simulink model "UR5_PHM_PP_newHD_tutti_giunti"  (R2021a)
settings: Solver=ode14x  StartTime=0.0  StopTime=Sim.time  FixedStep=Sim.dt  MaxStep=Sim.dt  RelTol=1e-3  EnableMultiTasking=on
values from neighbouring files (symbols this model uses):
  alpha_n = 0.98*pi/180    (= 0.0171042266695)    [parameters.m]
  alpha_t = 30*pi/180    (= 0.523598775598)    [parameters.m]
  alpha_TTS = 0    [parameters.m]
  alpha_Tw_L = -6.9e-4    (= -0.00069)    [parameters.m]
  alpha_Tw_R = 3.9e-3    (= 0.0039)    [parameters.m]
  Beta_TTS = 0    [parameters.m]
  c1 = 1e-2    (= 0.01)    [parameters.m]
  c2 = 1e-2    (= 0.01)    [parameters.m]
  c3 = 1e-2    (= 0.01)    [parameters.m]
  c4 = 1e-2    (= 0.01)    [parameters.m]
  c5 = 1e-2    (= 0.01)    [parameters.m]
  c6 = 1e-2    (= 0.01)    [parameters.m]
  Cb1 = 1.8e3    (= 1800)    [parameters.m]
  Cb2 = 1.8e3    (= 1800)    [parameters.m]
  Cb3 = 1.8e3    (= 1800)    [parameters.m]
  Cb4 = 1.8e3    (= 1800)    [parameters.m]
  Cb5 = 1.8e3    (= 1800)    [parameters.m]
  Cb6 = 1.8e3    (= 1800)    [parameters.m]
  Cth_housing = 153.90    (= 153.9)    [parameters.m]
  Cth_w = 74.20    (= 74.2)    [parameters.m]
  dt_PP = 0.05    [parameters.m]
  Fric1 = [fc_1/2 1e1 fc_1 fv_1]    [parameters.m]
  Fric2 = [fc_2/2 1e1 fc_2 fv_2]    [parameters.m]
  Fric3 = [fc_3/2 1e1 fc_3 fv_3]    [parameters.m]
  Fric4 = [fc_4/2 1e1 fc_4 fv_4]    [parameters.m]
  Fric5 = [fc_5/2 1e1 fc_5 fv_5]    [parameters.m]
  Fric6 = [fc_6/2 1e1 fc_6 fv_6]    [parameters.m]
  Hth_housing = 0.30    (= 0.3)    [parameters.m]
  Hth_w = 1.14    [parameters.m]
  I_actual = I_actual(1:10,:)    [trajcutting.m]
  J_CS1 = 7.12e-5    (= 7.12e-05)    [parameters.m]
  J_CS2 = 7.12e-5    (= 7.12e-05)    [parameters.m]
  J_CS3 = 7.12e-5    (= 7.12e-05)    [parameters.m]
  J_CS4 = 6e-6    (= 6e-06)    [parameters.m]
  J_CS5 = 6e-6    (= 6e-06)    [parameters.m]
  J_CS6 = 6e-6    (= 6e-06)    [parameters.m]
  J_FS1 = 1.62e-7    (= 1.62e-07)    [parameters.m]
  J_FS2 = 1.62e-7    (= 1.62e-07)    [parameters.m]
  J_FS3 = 1.62e-7    (= 1.62e-07)    [parameters.m]
  J_FS4 = 4.97e-8    (= 4.97e-08)    [parameters.m]
  J_FS5 = 4.97e-8    (= 4.97e-08)    [parameters.m]
  J_FS6 = 4.97e-8    (= 4.97e-08)    [parameters.m]
  J_WG1 = 3.56e-5    (= 3.56e-05)    [parameters.m]
  J_WG2 = 3.56e-5    (= 3.56e-05)    [parameters.m]
  J_WG3 = 3.56e-5    (= 3.56e-05)    [parameters.m]
  J_WG4 = 3e-6    (= 3e-06)    [parameters.m]
  J_WG5 = 3e-6    (= 3e-06)    [parameters.m]
  J_WG6 = 3e-6    (= 3e-06)    [parameters.m]
  K_i = 1    [parameters.m]
  K_p = 1    [parameters.m]
  K_torsCS1 = 4.78e6    (= 4780000)    [parameters.m]
  K_torsCS2 = 4.78e6    (= 4780000)    [parameters.m]
  K_torsCS3 = 4.78e6    (= 4780000)    [parameters.m]
  K_torsCS4 = 1.06e6    (= 1060000)    [parameters.m]
  K_torsCS5 = 1.06e6    (= 1060000)    [parameters.m]
  K_torsCS6 = 1.06e6    (= 1060000)    [parameters.m]
  K_torsWG1 = 9.56e5    (= 956000)    [parameters.m]
  K_torsWG2 = 9.56e5    (= 956000)    [parameters.m]
  K_torsWG3 = 9.56e5    (= 956000)    [parameters.m]
  K_torsWG4 = 1.84e5    (= 184000)    [parameters.m]
  K_torsWG5 = 1.84e5    (= 184000)    [parameters.m]
  K_torsWG6 = 1.84e5    (= 184000)    [parameters.m]
  K_v = 1    [parameters.m]
  Kb1 = 0.51e8    (= 51000000)    [parameters.m]
  Kb2 = 0.51e8    (= 51000000)    [parameters.m]
  Kb3 = 0.51e8    (= 51000000)    [parameters.m]
  Kb4 = 1.98e7    (= 19800000)    [parameters.m]
  Kb5 = 1.98e7    (= 19800000)    [parameters.m]
  Kb6 = 1.98e7    (= 19800000)    [parameters.m]
  Km1 = 1.2e9    (= 1200000000)    [parameters.m]
  Km2 = 1.2e9    (= 1200000000)    [parameters.m]
  Km3 = 1.2e9    (= 1200000000)    [parameters.m]
  Km4 = 5.55e8    (= 555000000)    [parameters.m]
  Km5 = 5.55e8    (= 555000000)    [parameters.m]
  Km6 = 5.55e8    (= 555000000)    [parameters.m]
  Kt1 = 0.96e5    (= 96000)    [parameters.m]
  Kt2 = 0.96e5    (= 96000)    [parameters.m]
  Kt3 = 0.96e5    (= 96000)    [parameters.m]
  Kt4 = 1.15e4    (= 11500)    [parameters.m]
  Kt5 = 1.15e4    (= 11500)    [parameters.m]
  Kt6 = 1.15e4    (= 11500)    [parameters.m]
  L = Motor.L_2/2    [parameters.m]
  m2 = polyfit(Temp(:,2),pBn_UR5_f_Temp(:,2),1)    [parameters.m]
  mb2 = polyfit(Temp(:,8),pBn_UR5_f_Temp(:,8),1)    [parameters.m]
  pickTime = t_pick(traj)    [parameters.m]
  placeTime = t_place(traj)    [parameters.m]
  q0 = q_target(1,:)    [testlaw_PP.m]
  q_CS01 = x(6)    [parameters.m]
  q_CS02 = x(6)    [parameters.m]
  q_CS03 = x(6)    [parameters.m]
  q_CS04 = x(6)    [parameters.m]
  q_CS05 = x(6)    [parameters.m]
  q_CS06 = x(6)    [parameters.m]
  q_WG01 = x(1)    [parameters.m]
  q_WG02 = x(1)    [parameters.m]
  q_WG03 = x(1)    [parameters.m]
  q_WG04 = x(1)    [parameters.m]
  q_WG05 = x(1)    [parameters.m]
  q_WG06 = x(1)    [parameters.m]
  quant_i = [Motor.imax1 Motor.imax2      Motor.imax3 Motor.imax4 Motor.imax5 Motor.imax6]/2^16    [parameters.m]
  R = Motor.R_2/2    [parameters.m]
  rg1 = 0.028    [parameters.m]
  rg2 = 0.028    [parameters.m]
  rg3 = 0.028    [parameters.m]
  rg4 = 0.0155    [parameters.m]
  rg5 = 0.0155    [parameters.m]
  rg6 = 0.0155    [parameters.m]
  sigma_p = 444.29    [parameters.m]
  sigma_v = 2*pi*1000    (= 6283.18530718)    [parameters.m]
  stiff_red = 1    [parameters.m]
  T_0 = Sim.temp    [parameters.m]
  T_switch = 1e-4    (= 0.0001)    [parameters.m]
  tau_i = 1/(fc_i*2*pi)    (= 7.95774715459e-05)    [parameters.m]
  U_s = 48    [parameters.m]
  var_i = 1e-1*[.0167 .0184 .0144 .0016      .0011 .0007]    [parameters.m]
  var_p = 1e-6*[.0943 .3877      .3478 .5436 .3400 .2081]    [parameters.m]
  var_v = 1e-4*[.0738 .1452      .1564 .4623 .1824 .0917]    [parameters.m]
  Wf_TTS_0 = 0    [parameters.m]
  Wf_TTS_ONOFF = 0    [parameters.m]
  x2_01 = x(3)    [parameters.m]
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undefined symbols (not defined in the file or in its folder): deg, Driver1, Driver2, Driver3, Driver4, Driver5, Driver6, elseif, geom, Ground, J1, J2, J3, J4, J5, J6, kg, L1, L2, L3, L4, L5, L6, LINK0, LINK1, LINK2, LINK3, LINK4, LINK5, LINK6, m, Motor, N, payload, ROBOTIQ_FT, s, Sim, Tool, X, Y, Z
libraries: sm_lib x35, nesl_utility x30, simulink x23, simulink_extras x11, spsTriangleGeneratorLib x6
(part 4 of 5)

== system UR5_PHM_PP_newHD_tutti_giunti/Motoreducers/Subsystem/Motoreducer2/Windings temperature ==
  note: Coupling
  note: Housing
  note: Windings
  note: W_joule
  W_joule [W] : Inport
  T_ext [°C] : Inport  Port=2
  Add : Sum  Inputs=-+
  Add1 : Sum  Inputs=+-
  Add2 : Sum  Inputs=+-
  Add3 : Sum  Inputs=-+
  Add4 : Sum  Inputs=+-
  Gain : Gain  Gain=Hth_housing
  Gain1 : Gain  Gain=1/Cth_w
  Gain2 : Gain  Gain=Hth_w
  Gain3 : Gain  Gain=1/Cth_housing
  Gain4 : Gain  Gain=Hth_housing
  Integrator : Integrator  InitialCondition=T_0  LimitOutput=on  LowerSaturationLimit=-273.15
  Integrator1 : Integrator  InitialCondition=T_0  LimitOutput=on  LowerSaturationLimit=-273.15
  Tw [°C] : Outport  VectorParamsAs1DForOutWhenUnconnected=off
  Th [°C] : Outport  Port=2
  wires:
  W_joule [W]/1 -> Add/2
  Add/1 -> Gain1/1
  Gain1/1 -> Integrator/1
  Gain2/1 -> Add/1
  Integrator/1 -> Add2/1, Add1/1, Tw [°C]/1  "Tw"
  Add2/1 -> Gain2/1
  Integrator1/1 -> Th [°C]/1, Add3/2, Add1/2, Add2/2  "Thouse"
  Gain3/1 -> Integrator1/1
  T_ext [°C]/1 -> Add3/1
  Add1/1 -> Gain/1
  Add3/1 -> Gain4/1
  Gain4/1 -> Add4/2
  Gain/1 -> Add4/1
  Add4/1 -> Gain3/1

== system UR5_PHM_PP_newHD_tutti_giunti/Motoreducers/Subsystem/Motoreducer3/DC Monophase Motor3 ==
  Vset : Inport
  C : Inport  Port=2
  Gain4 : Gain  Gain=1/Motor.Im_123
  Integrator : Integrator
  Integrator1 : Integrator  InitialCondition=q0(3)*Motor.tau
  Monophase - BLDC : Subsystem
  Mux : Mux  Inputs=3
  Sum : Sum  Inputs=|+-
  i : Outport
  qm,qdm,qddm : Outport  Port=2  VectorParamsAs1DForOutWhenUnconnected=off
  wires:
  Monophase - BLDC/2(i) -> i/1  "i_j3"
  Vset/1 -> Monophase - BLDC/1(Vset)
  Monophase - BLDC/1(T) -> Sum/1  "Tem_j3"
  Sum/1 -> Gain4/1  "Tem-C_j3"
  Gain4/1 -> Mux/3, Integrator/1
  Integrator/1 -> Monophase - BLDC/2(qdm), Mux/2, Integrator1/1
  Mux/1 -> qm,qdm,qddm/1
  Integrator1/1 -> Mux/1  "qm_j3"
  C/1 -> Sum/2  "C_j3"

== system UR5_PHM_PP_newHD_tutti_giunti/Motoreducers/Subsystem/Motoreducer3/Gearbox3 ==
  C : Inport
  qd : Inport  Port=2
  " eta" : Gain  Gain=Motor.eta
  Abs : Abs
  Abs2 : Abs
  Add2 : Sum  Inputs=+|-
  Friction Function1 : Fcn  Expr=Fric3(1)*(1-tanh(Fric3(2)*u)) + Fric3(3) + Fric3(4)*u
  MinMax2 : MinMax  Inputs=2
  Product : Product  RndMeth=Zero
  Saturation : Saturate  UpperLimit=150  LowerLimit=-150
  Sign : Signum
  Sign1 : Signum
  Switch : Switch  Criteria=u2 > Threshold  Threshold=0.0
  Switch1 : Switch  Criteria=u2 > Threshold  Threshold=0.5
  Zero Detection : Fcn  Expr=abs(u(1))<1e-6
  Tu : Outport  VectorParamsAs1DForOutWhenUnconnected=off
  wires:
  Friction Function1/1 -> MinMax2/2, Switch1/3
  Add2/1 -> Tu/1  "Transmitted torque [Nm]"
  Zero Detection/1 -> Switch/2, Switch1/2
  C/1 -> " eta"/1
  Sign1/1 -> Switch/3
  " eta"/1 -> Saturation/1
  Switch1/1 -> Product/2
  Abs2/1 -> Friction Function1/1
  Sign/1 -> Switch/1
  Product/1 -> Add2/2  "Passive torque [Nm]"
  Switch/1 -> Product/1
  qd/1 -> Zero Detection/1, Sign1/1, Abs2/1
  MinMax2/1 -> Switch1/1
  Abs/1 -> MinMax2/1
  Saturation/1 -> Sign/1, Abs/1, Add2/1

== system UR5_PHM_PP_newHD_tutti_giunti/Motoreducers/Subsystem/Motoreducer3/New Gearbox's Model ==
  Delta_q : Inport
  qm : Inport  Port=2
  qdm : Inport  Port=3
  Delta_qd : Inport  Port=4
  q : Inport  Port=5
  qd : Inport  Port=6
  Abs : Abs
  Constant1 : Constant  Value=0
  Constant2 : Constant  Value=J3.clearance
  Constant3 : Constant  Value=J3.clearance
  Mux : Mux  Inputs=3
  No Backlash : Subsystem  TreatAsAtomicUnit=on
  No contact : Subsystem  Commented=on  TreatAsAtomicUnit=on
  Scope : Scope
  "if Height < Max low altitude elseif Height > Min isotropic altitude " : If  NumInputs=4  IfExpression=u1<=1e-10  ElseIfExpressions=u2>u3, u2<u4
  phi diff > max backlash : Subsystem  Commented=on  TreatAsAtomicUnit=on
  phi diff< min backlash : Subsystem  Commented=on  TreatAsAtomicUnit=on
  C1 : Outport
  Tu : Outport  Port=2  VectorParamsAs1DForOutWhenUnconnected=off
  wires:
  Constant3/1 -> Abs/1
  [Vel_rel] -> No contact/2(In3)
  [Pos_rel] -> No contact/1(In2)
  No contact/1(Out3) -> ?
  [ELSE] -> No contact/Action
  phi diff< min backlash/1(Out1) -> ?
  phi diff > max backlash/1(Out1) -> ?
  [Pos_rel] -> phi diff< min backlash/1(In2)
  [Vel_rel] -> phi diff< min backlash/2(In3)
  [ELSEIF2] -> phi diff< min backlash/Action
  [Pos_rel] -> phi diff > max backlash/1(In2)
  [Vel_rel] -> phi diff > max backlash/2(In3)
  [IF] -> No Backlash/Action
  [ELSEIF1] -> phi diff > max backlash/Action
  "if Height < Max low altitude elseif Height > Min isotropic altitude "/3 -> [ELSEIF2]
  Constant1/1 -> Mux/3, "if Height < Max low altitude elseif Height > Min isotropic altitude "/4
  Constant2/1 -> Mux/2, "if Height < Max low altitude elseif Height > Min isotropic altitude "/3
  Abs/1 -> "if Height < Max low altitude elseif Height > Min isotropic altitude "/1
  "if Height < Max low altitude elseif Height > Min isotropic altitude "/4 -> [ELSE]
  "if Height < Max low altitude elseif Height > Min isotropic altitude "/2 -> [ELSEIF1]
  "if Height < Max low altitude elseif Height > Min isotropic altitude "/1 -> [IF]
  Delta_q/1 -> Mux/1, "if Height < Max low altitude elseif Height > Min isotropic altitude "/2, [Pos_rel]
  Mux/1 -> Scope/1
  Delta_qd/1 -> [Vel_rel]
  No Backlash/1(Ccs->giunto) -> Tu/1
  q/1 -> No Backlash/2(q)
  qm/1 -> No Backlash/1(qm)
  qdm/1 -> No Backlash/3(qdm)
  qd/1 -> No Backlash/4(qd)
  No Backlash/2(Cwg->rotore) -> C1/1

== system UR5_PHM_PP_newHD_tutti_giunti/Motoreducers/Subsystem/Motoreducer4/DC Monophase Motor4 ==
  Vset : Inport
  C : Inport  Port=2
  Gain4 : Gain  Gain=1/Motor.Im_456
  Integrator : Integrator
  Integrator1 : Integrator  InitialCondition=q0(4)*Motor.tau
  Monophase - BLDC : Subsystem
  Mux : Mux  Inputs=3
  Sum : Sum  Inputs=|+-
  i : Outport
  qm,qdm,qddm : Outport  Port=2  VectorParamsAs1DForOutWhenUnconnected=off
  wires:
  Monophase - BLDC/2(i) -> i/1  "i_j4"
  Vset/1 -> Monophase - BLDC/1(Vset)
  Monophase - BLDC/1(T) -> Sum/1  "Tem_j4"
  Sum/1 -> Gain4/1  "Tem-C_j4"
  Gain4/1 -> Mux/3, Integrator/1
  Integrator/1 -> Monophase - BLDC/2(qdm), Mux/2, Integrator1/1
  Mux/1 -> qm,qdm,qddm/1
  Integrator1/1 -> Mux/1  "qm_j4"
  C/1 -> Sum/2  "C_j4"

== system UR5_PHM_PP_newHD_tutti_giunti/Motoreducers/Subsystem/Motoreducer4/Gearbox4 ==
  C : Inport
  qd : Inport  Port=2
  " eta" : Gain  Gain=Motor.eta
  Abs : Abs
  Abs2 : Abs
  Add2 : Sum  Inputs=+|-
  Friction Function1 : Fcn  Expr=Fric4(1)*(1-tanh(Fric4(2)*u)) + Fric4(3) + Fric4(4)*u
  MinMax2 : MinMax  Inputs=2
  Product : Product  RndMeth=Zero
  Saturation : Saturate  UpperLimit=28  LowerLimit=-28
  Sign : Signum
  Sign1 : Signum
  Switch : Switch  Criteria=u2 > Threshold  Threshold=0.0
  Switch1 : Switch  Criteria=u2 > Threshold  Threshold=0.5
  Zero Detection : Fcn  Expr=abs(u(1))<1e-6
  Tu : Outport  VectorParamsAs1DForOutWhenUnconnected=off
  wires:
  Switch1/1 -> Product/2
  Sign/1 -> Switch/1
  Product/1 -> Add2/2  "Passive torque [Nm]"
  Switch/1 -> Product/1
  C/1 -> " eta"/1
  MinMax2/1 -> Switch1/1
  Sign1/1 -> Switch/3
  Add2/1 -> Tu/1  "Transmitted torque [Nm]"
  Abs/1 -> MinMax2/1
  " eta"/1 -> Saturation/1
  Abs2/1 -> Friction Function1/1
  Friction Function1/1 -> MinMax2/2, Switch1/3
  Zero Detection/1 -> Switch/2, Switch1/2
  qd/1 -> Zero Detection/1, Sign1/1, Abs2/1
  Saturation/1 -> Sign/1, Abs/1, Add2/1

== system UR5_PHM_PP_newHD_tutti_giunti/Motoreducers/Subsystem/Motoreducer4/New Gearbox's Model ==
  Delta_q : Inport
  qm : Inport  Port=2
  qdm : Inport  Port=3
  Delta_qd : Inport  Port=4
  q : Inport  Port=5
  qd : Inport  Port=6
  Abs : Abs
  Constant1 : Constant  Value=0
  Constant2 : Constant  Value=J4.clearance
  Constant3 : Constant  Value=J4.clearance
  Mux : Mux  Inputs=3
  No Backlash : Subsystem  TreatAsAtomicUnit=on
  No contact : Subsystem  Commented=on  TreatAsAtomicUnit=on
  Scope : Scope
  "if Height < Max low altitude elseif Height > Min isotropic altitude " : If  NumInputs=4  IfExpression=u1<=1e-10  ElseIfExpressions=u2>u3, u2<u4
  phi diff > max backlash : Subsystem  Commented=on  TreatAsAtomicUnit=on
  phi diff< min backlash : Subsystem  Commented=on  TreatAsAtomicUnit=on
  C1 : Outport
  C2 : Outport  Port=2  VectorParamsAs1DForOutWhenUnconnected=off
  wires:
  Constant3/1 -> Abs/1
  [Vel_rel] -> No contact/2(In3)
  [Pos_rel] -> No contact/1(In2)
  No contact/1(Out3) -> ?
  [ELSE] -> No contact/Action
  phi diff< min backlash/1(Out1) -> ?
  phi diff > max backlash/1(Out1) -> ?
  [Pos_rel] -> phi diff< min backlash/1(In2)
  [Vel_rel] -> phi diff< min backlash/2(In3)
  [ELSEIF2] -> phi diff< min backlash/Action
  [Pos_rel] -> phi diff > max backlash/1(In2)
  [Vel_rel] -> phi diff > max backlash/2(In3)
  [IF] -> No Backlash/Action
  [ELSEIF1] -> phi diff > max backlash/Action
  "if Height < Max low altitude elseif Height > Min isotropic altitude "/3 -> [ELSEIF2]
  Constant1/1 -> Mux/3, "if Height < Max low altitude elseif Height > Min isotropic altitude "/4
  Constant2/1 -> Mux/2, "if Height < Max low altitude elseif Height > Min isotropic altitude "/3
  Abs/1 -> "if Height < Max low altitude elseif Height > Min isotropic altitude "/1
  "if Height < Max low altitude elseif Height > Min isotropic altitude "/4 -> [ELSE]
  "if Height < Max low altitude elseif Height > Min isotropic altitude "/2 -> [ELSEIF1]
  "if Height < Max low altitude elseif Height > Min isotropic altitude "/1 -> [IF]
  Delta_q/1 -> Mux/1, "if Height < Max low altitude elseif Height > Min isotropic altitude "/2, [Pos_rel]
  Mux/1 -> Scope/1
  Delta_qd/1 -> [Vel_rel]
  qm/1 -> No Backlash/1(qm)
  q/1 -> No Backlash/2(q)
  qdm/1 -> No Backlash/3(qdm)
  qd/1 -> No Backlash/4(qd)
  No Backlash/1(Ccs->giunto) -> C2/1
  No Backlash/2(Cwg->rotore) -> C1/1

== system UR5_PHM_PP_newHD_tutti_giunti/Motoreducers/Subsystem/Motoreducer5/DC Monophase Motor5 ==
  Vset : Inport
  C : Inport  Port=2
  Gain4 : Gain  Gain=1/Motor.Im_456
  Integrator : Integrator
  Integrator1 : Integrator  InitialCondition=q0(5)*Motor.tau
  Monophase - BLDC : Subsystem
  Mux : Mux  Inputs=3
  Sum : Sum  Inputs=|+-
  i : Outport
  qm,qdm,qddm : Outport  Port=2  VectorParamsAs1DForOutWhenUnconnected=off
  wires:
  Monophase - BLDC/2(i) -> i/1  "i_j5"
  Vset/1 -> Monophase - BLDC/1(Vset)
  Monophase - BLDC/1(T) -> Sum/1  "Tem_j5"
  Sum/1 -> Gain4/1  "Tem-C_j5"
  Gain4/1 -> Mux/3, Integrator/1
  Integrator/1 -> Monophase - BLDC/2(qdm), Mux/2, Integrator1/1
  Mux/1 -> qm,qdm,qddm/1
  Integrator1/1 -> Mux/1  "qm_j5"
  C/1 -> Sum/2  "C_j5"

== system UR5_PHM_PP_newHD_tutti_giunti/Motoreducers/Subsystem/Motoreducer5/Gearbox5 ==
  C : Inport
  qd : Inport  Port=2
  Abs : Abs
  Abs2 : Abs
  Add2 : Sum  Inputs=+|-
  Friction Function1 : Fcn  Expr=Fric5(1)*(1-tanh(Fric5(2)*u)) + Fric5(3) + Fric5(4)*u
  MinMax2 : MinMax  Inputs=2
  Product : Product  RndMeth=Zero
  Saturation : Saturate  UpperLimit=28  LowerLimit=-28
  Sign : Signum
  Sign1 : Signum
  Switch : Switch  Criteria=u2 > Threshold  Threshold=0.0
  Switch1 : Switch  Criteria=u2 > Threshold  Threshold=0.5
  Zero Detection : Fcn  Expr=abs(u(1))<1e-6
  eta : Gain  Gain=Motor.eta
  Tu : Outport  VectorParamsAs1DForOutWhenUnconnected=off
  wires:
  qd/1 -> Zero Detection/1, Sign1/1, Abs2/1
  Sign1/1 -> Switch/3
  Friction Function1/1 -> MinMax2/2, Switch1/3
  Abs2/1 -> Friction Function1/1
  eta/1 -> Saturation/1
  Add2/1 -> Tu/1  "Transmitted torque [Nm]"
  C/1 -> eta/1
  Switch1/1 -> Product/2
  Switch/1 -> Product/1
  Abs/1 -> MinMax2/1
  MinMax2/1 -> Switch1/1
  Sign/1 -> Switch/1
  Zero Detection/1 -> Switch/2, Switch1/2
  Product/1 -> Add2/2  "Passive torque [Nm]"
  Saturation/1 -> Sign/1, Abs/1, Add2/1

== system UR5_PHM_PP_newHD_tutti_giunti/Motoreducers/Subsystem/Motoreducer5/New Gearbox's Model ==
  Delta_q : Inport
  qm : Inport  Port=2
  qdm : Inport  Port=3
  Delta_qd : Inport  Port=4
  q : Inport  Port=5
  qd : Inport  Port=6
  Abs : Abs
  Constant1 : Constant  Value=0
  Constant2 : Constant  Value=J5.clearance
  Constant3 : Constant  Value=J5.clearance
  Mux : Mux  Inputs=3
  No Backlash : Subsystem  TreatAsAtomicUnit=on
  No contact : Subsystem  Commented=on  TreatAsAtomicUnit=on
  Scope : Scope
  "if Height < Max low altitude elseif Height > Min isotropic altitude " : If  NumInputs=4  IfExpression=u1<=1e-10  ElseIfExpressions=u2>u3, u2<u4
  phi diff > max backlash : Subsystem  Commented=on  TreatAsAtomicUnit=on
  phi diff< min backlash : Subsystem  Commented=on  TreatAsAtomicUnit=on
  C1 : Outport
  C2 : Outport  Port=2  VectorParamsAs1DForOutWhenUnconnected=off
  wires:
  Constant3/1 -> Abs/1
  [Vel_rel] -> No contact/2(In3)
  [Pos_rel] -> No contact/1(In2)
  No contact/1(Out3) -> ?
  [ELSE] -> No contact/Action
  phi diff< min backlash/1(Out1) -> ?
  phi diff > max backlash/1(Out1) -> ?
  [Pos_rel] -> phi diff< min backlash/1(In2)
  [Vel_rel] -> phi diff< min backlash/2(In3)
  [ELSEIF2] -> phi diff< min backlash/Action
  [Pos_rel] -> phi diff > max backlash/1(In2)
  [Vel_rel] -> phi diff > max backlash/2(In3)
  [IF] -> No Backlash/Action
  [ELSEIF1] -> phi diff > max backlash/Action
  "if Height < Max low altitude elseif Height > Min isotropic altitude "/3 -> [ELSEIF2]
  Constant1/1 -> Mux/3, "if Height < Max low altitude elseif Height > Min isotropic altitude "/4
  Constant2/1 -> Mux/2, "if Height < Max low altitude elseif Height > Min isotropic altitude "/3
  Abs/1 -> "if Height < Max low altitude elseif Height > Min isotropic altitude "/1
  "if Height < Max low altitude elseif Height > Min isotropic altitude "/4 -> [ELSE]
  "if Height < Max low altitude elseif Height > Min isotropic altitude "/2 -> [ELSEIF1]
  "if Height < Max low altitude elseif Height > Min isotropic altitude "/1 -> [IF]
  Delta_q/1 -> Mux/1, "if Height < Max low altitude elseif Height > Min isotropic altitude "/2, [Pos_rel]
  Mux/1 -> Scope/1
  Delta_qd/1 -> [Vel_rel]
  qm/1 -> No Backlash/1(qm)
  q/1 -> No Backlash/2(q)
  qdm/1 -> No Backlash/3(qdm)
  qd/1 -> No Backlash/4(qd)
  No Backlash/1(Ccs->giunto) -> C2/1
  No Backlash/2(Cwg->rotore) -> C1/1

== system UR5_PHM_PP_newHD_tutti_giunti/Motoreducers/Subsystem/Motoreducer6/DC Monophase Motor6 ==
  Vset : Inport
  C : Inport  Port=2
  Gain4 : Gain  Gain=1/Motor.Im_456
  Integrator : Integrator
  Integrator1 : Integrator  InitialCondition=q0(6)*Motor.tau
  Monophase - BLDC : Subsystem
  Mux : Mux  Inputs=3
  Sum : Sum  Inputs=|+-
  i : Outport
  qm,qdm,qddm : Outport  Port=2  VectorParamsAs1DForOutWhenUnconnected=off
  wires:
  Monophase - BLDC/2(i) -> i/1  "i_j6"
  Vset/1 -> Monophase - BLDC/1(Vset)
  Monophase - BLDC/1(T) -> Sum/1  "Tem_j6"
  Sum/1 -> Gain4/1  "Tem-C_j6"
  Gain4/1 -> Mux/3, Integrator/1
  Integrator/1 -> Monophase - BLDC/2(qdm), Mux/2, Integrator1/1
  Mux/1 -> qm,qdm,qddm/1
  Integrator1/1 -> Mux/1  "qm_j6"
  C/1 -> Sum/2  "C_j6"

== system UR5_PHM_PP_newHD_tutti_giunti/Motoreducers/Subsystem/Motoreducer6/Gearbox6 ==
  C : Inport
  qd : Inport  Port=2
  " eta" : Gain  Gain=Motor.eta
  Abs : Abs
  Abs2 : Abs
  Add2 : Sum  Inputs=+|-
  Friction Function1 : Fcn  Expr=Fric6(1)*(1-tanh(Fric6(2)*u)) + Fric6(3) + Fric6(4)*u
  MinMax2 : MinMax  Inputs=2
  Product : Product  RndMeth=Zero
  Saturation : Saturate  UpperLimit=28  LowerLimit=-28
  Sign : Signum
  Sign1 : Signum
  Switch : Switch  Criteria=u2 > Threshold  Threshold=0.0
  Switch1 : Switch  Criteria=u2 > Threshold  Threshold=0.5
  Zero Detection : Fcn  Expr=abs(u(1))<1e-6
  Tu : Outport  VectorParamsAs1DForOutWhenUnconnected=off
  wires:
  Add2/1 -> Tu/1  "Transmitted torque [Nm]"
  MinMax2/1 -> Switch1/1
  Sign/1 -> Switch/1
  Abs2/1 -> Friction Function1/1
  C/1 -> " eta"/1
  qd/1 -> Zero Detection/1, Sign1/1, Abs2/1
  Switch/1 -> Product/1
  " eta"/1 -> Saturation/1
  Abs/1 -> MinMax2/1
  Friction Function1/1 -> MinMax2/2, Switch1/3
  Zero Detection/1 -> Switch/2, Switch1/2
  Switch1/1 -> Product/2
  Sign1/1 -> Switch/3
  Product/1 -> Add2/2  "Passive torque [Nm]"
  Saturation/1 -> Sign/1, Abs/1, Add2/1

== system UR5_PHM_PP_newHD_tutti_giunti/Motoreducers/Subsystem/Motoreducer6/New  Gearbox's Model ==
  Delta_q : Inport
  qm : Inport  Port=2
  qdm : Inport  Port=3
  Delta_qd : Inport  Port=4
  q : Inport  Port=5
  qd : Inport  Port=6
  Abs : Abs
  Constant1 : Constant  Value=0
  Constant2 : Constant  Value=J6.clearance
  Constant3 : Constant  Value=J6.clearance
  Mux : Mux  Inputs=3
  No Backlash : Subsystem  TreatAsAtomicUnit=on
  No contact : Subsystem  Commented=on  TreatAsAtomicUnit=on
  Scope : Scope
  "if Height < Max low altitude elseif Height > Min isotropic altitude " : If  NumInputs=4  IfExpression=u1<=1e-10  ElseIfExpressions=u2>u3, u2<u4
  phi diff > max backlash : Subsystem  Commented=on  TreatAsAtomicUnit=on
  phi diff< min backlash : Subsystem  Commented=on  TreatAsAtomicUnit=on
  C1 : Outport
  C2 : Outport  Port=2  VectorParamsAs1DForOutWhenUnconnected=off
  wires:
  Constant3/1 -> Abs/1
  [Vel_rel] -> No contact/2(In3)
  [Pos_rel] -> No contact/1(In2)
  No contact/1(Out3) -> ?
  [ELSE] -> No contact/Action
  phi diff< min backlash/1(Out1) -> ?
  phi diff > max backlash/1(Out1) -> ?
  [Pos_rel] -> phi diff< min backlash/1(In2)
  [Vel_rel] -> phi diff< min backlash/2(In3)
  [ELSEIF2] -> phi diff< min backlash/Action
  [Pos_rel] -> phi diff > max backlash/1(In2)
  [Vel_rel] -> phi diff > max backlash/2(In3)
  [IF] -> No Backlash/Action
  [ELSEIF1] -> phi diff > max backlash/Action
  "if Height < Max low altitude elseif Height > Min isotropic altitude "/3 -> [ELSEIF2]
  Constant1/1 -> Mux/3, "if Height < Max low altitude elseif Height > Min isotropic altitude "/4
  Constant2/1 -> Mux/2, "if Height < Max low altitude elseif Height > Min isotropic altitude "/3
  Abs/1 -> "if Height < Max low altitude elseif Height > Min isotropic altitude "/1
  "if Height < Max low altitude elseif Height > Min isotropic altitude "/4 -> [ELSE]
  "if Height < Max low altitude elseif Height > Min isotropic altitude "/2 -> [ELSEIF1]
  "if Height < Max low altitude elseif Height > Min isotropic altitude "/1 -> [IF]
  Delta_q/1 -> Mux/1, "if Height < Max low altitude elseif Height > Min isotropic altitude "/2, [Pos_rel]
  Mux/1 -> Scope/1
  Delta_qd/1 -> [Vel_rel]
  No Backlash/1(Ccs->giunto) -> C2/1
  qm/1 -> No Backlash/1(qm)
  q/1 -> No Backlash/2(q)
  qdm/1 -> No Backlash/3(qdm)
  qd/1 -> No Backlash/4(qd)
  No Backlash/2(Cwg->rotore) -> C1/1

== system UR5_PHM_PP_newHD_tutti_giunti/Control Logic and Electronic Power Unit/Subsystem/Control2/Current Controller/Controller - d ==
  id : Inport
  Add : Sum
  Add1 : Sum  Inputs=+-
  Constant : Constant  Value=0
  Integrator : Integrator
  ki_id : Gain  Gain=Driver2.Iid
  kp_id : Gain  Gain=Driver2.Pid
  saturation : Saturate  UpperLimit=52.11  LowerLimit=-52.11
  v*d : Outport  VectorParamsAs1DForOutWhenUnconnected=off
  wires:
  id/1 -> Add1/2
  Constant/1 -> Add1/1
  Integrator/1 -> Add/2
  kp_id/1 -> Add/1
  saturation/1 -> v*d/1
  Add1/1 -> ki_id/1, kp_id/1
  Add/1 -> saturation/1
  ki_id/1 -> Integrator/1

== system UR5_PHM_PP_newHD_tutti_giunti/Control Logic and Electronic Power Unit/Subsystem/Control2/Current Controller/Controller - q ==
  i* : Inport
  Iq : Inport  Port=2
  Add : Sum
  Add1 : Sum  Inputs=+-
  Integrator : Integrator
  ki_iq : Gain  Gain=Driver2.Iiq
  kp_iq : Gain  Gain=Driver2.Piq
  saturation : Saturate  UpperLimit=52.11  LowerLimit=-52.11
  v*q : Outport  VectorParamsAs1DForOutWhenUnconnected=off
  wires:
  Iq/1 -> Add1/2
  i*/1 -> Add1/1
  kp_iq/1 -> Add/1
  Add1/1 -> ki_iq/1, kp_iq/1
  Integrator/1 -> Add/2
  Add/1 -> saturation/1
  saturation/1 -> v*q/1
  ki_iq/1 -> Integrator/1

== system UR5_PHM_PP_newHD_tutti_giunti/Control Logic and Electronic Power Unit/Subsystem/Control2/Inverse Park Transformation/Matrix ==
  A11 : Inport
  A12 : Inport  Port=2
  A13 : Inport  Port=3
  A21 : Inport  Port=4
  A22 : Inport  Port=5
  A23 : Inport  Port=6
  A31 : Inport  Port=7
  A32 : Inport  Port=8
  A33 : Inport  Port=9
  Reshape : Reshape  OutputDimensionality=Customize  OutputDimensions=[3,3]
  Vector Concatenate : Concatenate  NumInputs=9
  Out1 : Outport  VectorParamsAs1DForOutWhenUnconnected=off
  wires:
  Vector Concatenate/1 -> Reshape/1
  A11/1 -> Vector Concatenate/1
  Reshape/1 -> Out1/1
  A22/1 -> Vector Concatenate/5
  A33/1 -> Vector Concatenate/9
  A21/1 -> Vector Concatenate/2
  A31/1 -> Vector Concatenate/3
  A12/1 -> Vector Concatenate/4
  A32/1 -> Vector Concatenate/6
  A13/1 -> Vector Concatenate/7
  A23/1 -> Vector Concatenate/8

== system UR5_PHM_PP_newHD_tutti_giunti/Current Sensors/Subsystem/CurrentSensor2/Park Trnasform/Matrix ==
  A11 : Inport
  A12 : Inport  Port=2
  A13 : Inport  Port=3
  A21 : Inport  Port=4
  A22 : Inport  Port=5
  A23 : Inport  Port=6
  A31 : Inport  Port=7
  A32 : Inport  Port=8
  A33 : Inport  Port=9
  Reshape : Reshape  OutputDimensionality=Customize  OutputDimensions=[3,3]
  Vector Concatenate : Concatenate  NumInputs=9
  Out1 : Outport  VectorParamsAs1DForOutWhenUnconnected=off
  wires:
  Vector Concatenate/1 -> Reshape/1
  A11/1 -> Vector Concatenate/1
  Reshape/1 -> Out1/1
  A22/1 -> Vector Concatenate/5
  A33/1 -> Vector Concatenate/9
  A21/1 -> Vector Concatenate/2
  A31/1 -> Vector Concatenate/3
  A12/1 -> Vector Concatenate/4
  A32/1 -> Vector Concatenate/6
  A13/1 -> Vector Concatenate/7
  A23/1 -> Vector Concatenate/8

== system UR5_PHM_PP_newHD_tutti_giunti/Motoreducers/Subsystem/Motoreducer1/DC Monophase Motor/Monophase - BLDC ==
  Vset : Inport
  qdm : Inport  Port=2
  Phase A : Subsystem
  Torque constant [Nm/A] : Gain  Gain=Motor.kc_1
  T : Outport  VectorParamsAs1DForOutWhenUnconnected=off
  i : Outport  Port=2  VectorParamsAs1DForOutWhenUnconnected=off
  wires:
  Vset/1 -> Phase A/1(Vset)
  Torque constant [Nm/A]/1 -> T/1
  Phase A/1(i) -> Torque constant [Nm/A]/1, i/1
  qdm/1 -> Phase A/2(qdm)

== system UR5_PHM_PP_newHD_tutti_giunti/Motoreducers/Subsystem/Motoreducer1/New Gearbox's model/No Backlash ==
  qm : Inport
  q : Inport  Port=2
  qdm : Inport  Port=3
  qd : Inport  Port=4
  Action Port : ActionPort  PropagateVarSize=During execution  ActionPortLabel=if(u1<=1e-10)
  Circular spline : Subsystem
  Flexspline (rad) : Subsystem
  Flexspline (tang) : Subsystem
  Wave Generator : Subsystem
  Ccs->giunto : Outport
  Cwg->rotore : Outport  Port=2
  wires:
  Flexspline (tang)/1(y1) -> Circular spline/3(y1), Flexspline (rad)/4(y1)
  Flexspline (rad)/1(y2) -> Flexspline (tang)/1(y2), Circular spline/1(y2)
  Flexspline (rad)/2(x2) -> Flexspline (tang)/2(x2), Circular spline/2(x2)
  q/1 -> Circular spline/4(q)
  qd/1 -> Circular spline/5(qd)
  Circular spline/2(q_CS) -> Flexspline (rad)/3(q_CS)
  Circular spline/1(C1) -> Ccs->giunto/1
  qm/1 -> Wave Generator/1(qm)
  qdm/1 -> Wave Generator/2(qdm)
  Flexspline (rad)/3(C_FS->WG) -> Wave Generator/3(C_FS->WG)
  Wave Generator/1(Cwg->rotore) -> Cwg->rotore/1
  Wave Generator/2(qm_WG) -> Flexspline (rad)/1(qm_WG)
  Wave Generator/3(qdm_WG) -> Flexspline (rad)/2(qdm_WG)

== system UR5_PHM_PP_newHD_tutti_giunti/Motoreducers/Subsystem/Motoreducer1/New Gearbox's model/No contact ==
  In2 : Inport
  In3 : Inport  Port=2
  Action Port : ActionPort  PropagateVarSize=During execution  ActionPortLabel=else
  1/(2-1/eta_dir) : Gain  Gain=0
  Add4 : Sum  Inputs=+|+
  Out3 : Outport  VectorParamsAs1DForOutWhenUnconnected=off
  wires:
  Add4/1 -> 1/(2-1/eta_dir)/1
  In3/1 -> Add4/2
  In2/1 -> Add4/1
  1/(2-1/eta_dir)/1 -> Out3/1

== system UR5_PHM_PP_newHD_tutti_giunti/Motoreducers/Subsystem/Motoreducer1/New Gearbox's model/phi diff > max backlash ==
  In2 : Inport
  In3 : Inport  Port=2
  Action Port : ActionPort  PropagateVarSize=During execution  ActionPortLabel=elseif(u2>u3)
  Add1 : Sum  Inputs=+|-
  Add2 : Sum  Inputs=+|+
  Add4 : Sum  Inputs=+|+
  Compare To Zero : simulink/Logic and Bit Operations/Compare To Zero  relop=<=  OutDataTypeStr=uint8
  Constant : Constant  Value=0
  Constant3 : Constant  Value=J1.clearance
  Cs_shaft [Nm/(rad/s)] : Gain  Gain=J1.C
  Ks_shaft [Nm/rad] : Gain  Gain=J1.K
  MinMax : MinMax  Inputs=2
  Switch : Switch  Criteria=u2 > Threshold
  Out1 : Outport  VectorParamsAs1DForOutWhenUnconnected=off
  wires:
  Switch/1 -> Out1/1
  Add2/1 -> Switch/3
  MinMax/1 -> Add2/2
  Add4/1 -> Compare To Zero/1
  Constant/1 -> Switch/1
  Compare To Zero/1 -> Switch/2
  Add1/1 -> Ks_shaft [Nm/rad]/1
  Constant3/1 -> Add1/2
  In2/1 -> Add1/1
  In3/1 -> Cs_shaft [Nm/(rad/s)]/1
  Cs_shaft [Nm/(rad/s)]/1 -> MinMax/2, Add4/2
  Ks_shaft [Nm/rad]/1 -> Add2/1, MinMax/1, Add4/1

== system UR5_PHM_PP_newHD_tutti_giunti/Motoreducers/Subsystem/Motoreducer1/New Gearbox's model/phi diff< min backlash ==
  In2 : Inport
  In3 : Inport  Port=2
  Action Port : ActionPort  PropagateVarSize=During execution  ActionPortLabel=elseif( u2<u4)
  Add1 : Sum  Inputs=+|-
  Add2 : Sum  Inputs=+|+
  Add4 : Sum  Inputs=+|+
  Compare To Zero : simulink/Logic and Bit Operations/Compare To Zero  relop=>=  OutDataTypeStr=uint8
  Constant : Constant  Value=0
  Constant1 : Constant  Value=0
  Cs_shaft [Nm/(rad/s)] : Gain  Gain=J1.C
  Ks_shaft [Nm/rad] : Gain  Gain=J1.K
  MinMax : MinMax  Function=max  Inputs=2
  Switch : Switch  Criteria=u2 > Threshold
  Out1 : Outport  VectorParamsAs1DForOutWhenUnconnected=off
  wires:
  Switch/1 -> Out1/1
  Add2/1 -> Switch/3
  MinMax/1 -> Add2/2
  Add4/1 -> Compare To Zero/1
  Constant/1 -> Switch/1
  Compare To Zero/1 -> Switch/2
  Add1/1 -> Ks_shaft [Nm/rad]/1
  Constant1/1 -> Add1/2
  In2/1 -> Add1/1
  In3/1 -> Cs_shaft [Nm/(rad/s)]/1
  Cs_shaft [Nm/(rad/s)]/1 -> MinMax/2, Add4/2
  Ks_shaft [Nm/rad]/1 -> Add2/1, MinMax/1, Add4/1

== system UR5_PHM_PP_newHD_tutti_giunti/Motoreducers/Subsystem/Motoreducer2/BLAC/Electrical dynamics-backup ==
  V[ao,bo,co] : Inport
  e[a,b,c] : Inport  Port=2
  T_W [*C] : Inport  Port=3
  Add{1..2,4,7} (4 alike) : Sum  Inputs=+-
  Demux : Demux  Outputs=3
  Demux1 : Demux  Outputs=3
  Divide : Product  Inputs=*/
  Integrator4 : Integrator  LimitOutput=on  UpperSaturationLimit=Motor.imax2  LowerSaturationLimit=-Motor.imax2
  Multiply : Product
  Multiply1 : Product
  Mux1 : Mux  Inputs=3
  "R,L, computation" : Subsystem
  Scope1 : Scope
  Scope2 : Scope
  Sum of Elements : Sum  Inputs=+
  i[a,b,c] : Outport  VectorParamsAs1DForOutWhenUnconnected=off
  W_joule[W] : Outport  Port=2  VectorParamsAs1DForOutWhenUnconnected=off
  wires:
  V[ao,bo,co]/1 -> Demux/1
  Demux/1 -> [Vao]  "Vao_j2"
  Demux/2 -> [Vbo]  "Vbo_j2"
  Demux/3 -> [Vco]  "Vco_j2"
  e[a,b,c]/1 -> Demux1/1
  Demux1/1 -> [ea]
  Demux1/2 -> [eb]
  Demux1/3 -> [ec]
  [ec] -> Add2/2
  Add2/1 -> Mux1/3
  [Vao] -> Add1/1
  [Vbo] -> Add4/1
  [Vco] -> Add2/1
  [ea] -> Add1/2
  Add4/1 -> Mux1/2
  [eb] -> Add4/2
  Add1/1 -> Mux1/1
  T_W [*C]/1 -> "R,L, computation"/1(Tw [°C])
  Divide/1 -> Integrator4/1
  Mux1/1 -> Add7/1
  Multiply/1 -> Multiply1/2, Add7/2
  Integrator4/1 -> Multiply1/1, Multiply/2, i[a,b,c]/1
  Add7/1 -> Divide/1
  "R,L, computation"/1(L[a,b,c]) -> Divide/2, Scope2/1  "L_j2"
  "R,L, computation"/2(R[a,b,c]) -> Scope1/1, Multiply/1  "R_j2"
  Multiply1/1 -> Sum of Elements/1
  Sum of Elements/1 -> W_joule[W]/1

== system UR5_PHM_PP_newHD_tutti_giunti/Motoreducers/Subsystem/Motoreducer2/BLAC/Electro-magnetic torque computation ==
  i[a,b,c] : Inport
  e[a,b,c]/theta_dot : Inport  Port=2
  Multiply : Product
  Scope : Scope  NumInputPorts=2
  Sum of Elements : Sum  Inputs=+
  Tem : Outport  VectorParamsAs1DForOutWhenUnconnected=off
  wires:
  e[a,b,c]/theta_dot/1 -> Scope/2, Multiply/2  "e_abc/qmd"
  i[a,b,c]/1 -> Scope/1, Multiply/1  "i_abc"
  Sum of Elements/1 -> Tem/1
  Multiply/1 -> Sum of Elements/1

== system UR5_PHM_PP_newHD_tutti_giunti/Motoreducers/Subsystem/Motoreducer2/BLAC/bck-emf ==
  qm : Inport
  qmd : Inport  Port=2
  Fcn : Fcn  Expr=cos(u(1))
  Fcn1 : Fcn  Expr=cos(u(1)-2/3*pi)
  Fcn2 : Fcn  Expr=cos(u(1)+2/3*pi)
  Gain : Gain  Gain=Motor.kv_2
  Gain1 : Gain  Gain=Motor.Zp_2
  Gain2 : Gain  Gain=Motor.kv_2
  Gain3 : Gain  Gain=Motor.kv_2
  Mux1 : Mux  Inputs=3
  Product3 : Product
  e[a,b,c] : Outport  VectorParamsAs1DForOutWhenUnconnected=off
  e[a,b,c]/theta_dot : Outport  Port=2  VectorParamsAs1DForOutWhenUnconnected=off
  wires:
  Fcn/1 -> Gain/1
  Gain/1 -> Mux1/1
  Product3/1 -> e[a,b,c]/1
  Mux1/1 -> Product3/2, e[a,b,c]/theta_dot/1
  qm/1 -> Gain1/1
  qmd/1 -> Product3/1
  Gain1/1 -> Fcn/1, Fcn1/1, Fcn2/1
  Fcn1/1 -> Gain2/1
  Gain2/1 -> Mux1/2
  Fcn2/1 -> Gain3/1
  Gain3/1 -> Mux1/3

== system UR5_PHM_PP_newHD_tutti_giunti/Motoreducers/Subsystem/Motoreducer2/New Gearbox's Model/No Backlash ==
  qm : Inport
  q : Inport  Port=2
  qdm : Inport  Port=3
  qd : Inport  Port=4
  Action Port : ActionPort  PropagateVarSize=During execution  ActionPortLabel=if(u1<=1e-10)
  Circular spline : Subsystem
  Flexspline (rad) : Subsystem
  Flexspline (tang) : Subsystem
  Wave Generator : Subsystem
  Ccs->giunto : Outport
  Cwg->rotore : Outport  Port=2
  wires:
  Flexspline (rad)/2(x2) -> Circular spline/3(x2), Flexspline (tang)/2(x2)
  Flexspline (rad)/1(y2) -> Circular spline/2(y2), Flexspline (tang)/1(y2)
  q/1 -> Circular spline/4(q)
  qd/1 -> Circular spline/5(qd)
  Circular spline/1(C1) -> Ccs->giunto/1
  Circular spline/2(q_CS) -> Flexspline (rad)/3(q_CS)
  qm/1 -> Wave Generator/1(qm)
  qdm/1 -> Wave Generator/2(qdm)
  Flexspline (rad)/3(C_FS->WG) -> Wave Generator/3(C_FS->WG)
  Wave Generator/1(C_wg->rotore) -> Cwg->rotore/1
  Wave Generator/2(qm_WG) -> Flexspline (rad)/1(qm_WG)
  Wave Generator/3(qdm_WG) -> Flexspline (rad)/2(qdm_WG)
  Flexspline (tang)/1(y1) -> Circular spline/1(y1), Flexspline (rad)/4(y1)

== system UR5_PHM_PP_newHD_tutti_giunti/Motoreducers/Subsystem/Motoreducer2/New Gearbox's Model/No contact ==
  In2 : Inport
  In3 : Inport  Port=2
  Action Port : ActionPort  PropagateVarSize=During execution  ActionPortLabel=else
  1/(2-1/eta_dir) : Gain  Gain=0
  Add4 : Sum  Inputs=+|+
  Out3 : Outport  VectorParamsAs1DForOutWhenUnconnected=off
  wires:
  Add4/1 -> 1/(2-1/eta_dir)/1
  In3/1 -> Add4/2
  In2/1 -> Add4/1
  1/(2-1/eta_dir)/1 -> Out3/1

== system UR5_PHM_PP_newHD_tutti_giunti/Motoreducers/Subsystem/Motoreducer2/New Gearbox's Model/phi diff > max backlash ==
  In2 : Inport
  In3 : Inport  Port=2
  Action Port : ActionPort  PropagateVarSize=During execution  ActionPortLabel=elseif(..)
  Add1 : Sum  Inputs=+|-
  Add2 : Sum  Inputs=+|+
  Add4 : Sum  Inputs=+|+
  Compare To Zero : simulink/Logic and Bit Operations/Compare To Zero  relop=<=  OutDataTypeStr=uint8
  Constant : Constant  Value=0
  Constant3 : Constant  Value=J2.clearance
  Cs_shaft [Nm/(rad/s)] : Gain  Gain=J2.C
  Ks_shaft [Nm/rad] : Gain  Gain=J2.K*stiff_red
  MinMax : MinMax  Inputs=2
  Switch : Switch  Criteria=u2 > Threshold
  Out1 : Outport  VectorParamsAs1DForOutWhenUnconnected=off
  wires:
  Switch/1 -> Out1/1
  Add2/1 -> Switch/3
  MinMax/1 -> Add2/2
  Add4/1 -> Compare To Zero/1
  Constant/1 -> Switch/1
  Compare To Zero/1 -> Switch/2
  Add1/1 -> Ks_shaft [Nm/rad]/1
  Constant3/1 -> Add1/2
  In2/1 -> Add1/1
  In3/1 -> Cs_shaft [Nm/(rad/s)]/1
  Cs_shaft [Nm/(rad/s)]/1 -> MinMax/2, Add4/2
  Ks_shaft [Nm/rad]/1 -> Add2/1, MinMax/1, Add4/1

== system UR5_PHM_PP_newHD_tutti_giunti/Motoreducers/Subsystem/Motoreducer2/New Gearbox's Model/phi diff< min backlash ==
  In2 : Inport
  In3 : Inport  Port=2
  Action Port : ActionPort  PropagateVarSize=During execution  ActionPortLabel=elseif(..)
  Add1 : Sum  Inputs=+|-
  Add2 : Sum  Inputs=+|+
  Add4 : Sum  Inputs=+|+
  Compare To Zero : simulink/Logic and Bit Operations/Compare To Zero  relop=>=  OutDataTypeStr=uint8
  Constant : Constant  Value=0
  Constant1 : Constant  Value=0
  Cs_shaft [Nm/(rad/s)] : Gain  Gain=J2.C
  Ks_shaft [Nm/rad] : Gain  Gain=J2.K*stiff_red
  MinMax : MinMax  Function=max  Inputs=2
  Switch : Switch  Criteria=u2 > Threshold
  Out1 : Outport  VectorParamsAs1DForOutWhenUnconnected=off
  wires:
  Switch/1 -> Out1/1
  Add2/1 -> Switch/3
  MinMax/1 -> Add2/2
  Add4/1 -> Compare To Zero/1
  Constant/1 -> Switch/1
  Compare To Zero/1 -> Switch/2
  Add1/1 -> Ks_shaft [Nm/rad]/1
  Constant1/1 -> Add1/2
  In2/1 -> Add1/1
  In3/1 -> Cs_shaft [Nm/(rad/s)]/1
  Cs_shaft [Nm/(rad/s)]/1 -> MinMax/2, Add4/2
  Ks_shaft [Nm/rad]/1 -> Add2/1, MinMax/1, Add4/1

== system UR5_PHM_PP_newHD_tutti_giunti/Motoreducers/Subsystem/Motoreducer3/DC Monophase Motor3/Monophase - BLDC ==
  Vset : Inport
  qdm : Inport  Port=2
  Phase A : Subsystem
  Torque constant [Nm/A] : Gain  Gain=Motor.kc_3
  T : Outport  VectorParamsAs1DForOutWhenUnconnected=off
  i : Outport  Port=2  VectorParamsAs1DForOutWhenUnconnected=off
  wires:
  Vset/1 -> Phase A/1(Vset)
  Torque constant [Nm/A]/1 -> T/1
  Phase A/1(i) -> Torque constant [Nm/A]/1, i/1
  qdm/1 -> Phase A/2(qdm)

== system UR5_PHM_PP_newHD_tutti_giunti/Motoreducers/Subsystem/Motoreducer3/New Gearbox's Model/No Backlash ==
  qm : Inport
  q : Inport  Port=2
  qdm : Inport  Port=3
  qd : Inport  Port=4
  Action Port : ActionPort  PropagateVarSize=During execution  ActionPortLabel=if(u1<=1e-10)
  Circular spline : Subsystem
  Flexspline (rad) : Subsystem
  Flexspline (tang) : Subsystem
  Wave Generator : Subsystem
  Ccs->giunto : Outport
  Cwg->rotore : Outport  Port=2
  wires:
  Flexspline (rad)/1(y2) -> Circular spline/2(y2), Flexspline (tang)/1(y2)
  Flexspline (rad)/2(x2) -> Circular spline/3(x2), Flexspline (tang)/2(x2)
  Flexspline (tang)/1(y1) -> Flexspline (rad)/4(y1), Circular spline/1(y1)
  q/1 -> Circular spline/4(q)
  qd/1 -> Circular spline/5(qd)
  Circular spline/1(C1) -> Ccs->giunto/1
  Circular spline/2(q_CS) -> Flexspline (rad)/3(q_CS)
  qm/1 -> Wave Generator/1(qm)
  qdm/1 -> Wave Generator/2(qdm)
  Flexspline (rad)/3(C_FS->WG) -> Wave Generator/3(C_FS->WG)
  Wave Generator/1(Cwg->rotore) -> Cwg->rotore/1
  Wave Generator/2(qm_WG) -> Flexspline (rad)/1(qm_WG)
  Wave Generator/3(qdm_WG) -> Flexspline (rad)/2(qdm_WG)

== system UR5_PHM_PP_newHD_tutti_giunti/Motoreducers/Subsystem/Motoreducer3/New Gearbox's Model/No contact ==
  In2 : Inport
  In3 : Inport  Port=2
  Action Port : ActionPort  PropagateVarSize=During execution  ActionPortLabel=else
  1/(2-1/eta_dir) : Gain  Gain=0
  Add4 : Sum  Inputs=+|+
  Out3 : Outport  VectorParamsAs1DForOutWhenUnconnected=off
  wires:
  Add4/1 -> 1/(2-1/eta_dir)/1
  In3/1 -> Add4/2
  In2/1 -> Add4/1
  1/(2-1/eta_dir)/1 -> Out3/1

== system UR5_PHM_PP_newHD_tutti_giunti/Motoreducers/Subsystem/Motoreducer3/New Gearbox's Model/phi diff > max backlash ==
  In2 : Inport
  In3 : Inport  Port=2
  Action Port : ActionPort  PropagateVarSize=During execution  ActionPortLabel=elseif(u2>u3)
  Add1 : Sum  Inputs=+|-
  Add2 : Sum  Inputs=+|+
  Add4 : Sum  Inputs=+|+
  Compare To Zero : simulink/Logic and Bit Operations/Compare To Zero  relop=<=  OutDataTypeStr=uint8
  Constant : Constant  Value=0
  Constant3 : Constant  Value=J1.clearance
  Cs_shaft [Nm/(rad/s)] : Gain  Gain=J3.C
  Ks_shaft [Nm/rad] : Gain  Gain=J3.K
  MinMax : MinMax  Inputs=2
  Switch : Switch  Criteria=u2 > Threshold
  Out1 : Outport  VectorParamsAs1DForOutWhenUnconnected=off
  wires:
  Switch/1 -> Out1/1
  Add2/1 -> Switch/3
  MinMax/1 -> Add2/2
  Add4/1 -> Compare To Zero/1
  Constant/1 -> Switch/1
  Compare To Zero/1 -> Switch/2
  Add1/1 -> Ks_shaft [Nm/rad]/1
  Constant3/1 -> Add1/2
  In2/1 -> Add1/1
  In3/1 -> Cs_shaft [Nm/(rad/s)]/1
  Cs_shaft [Nm/(rad/s)]/1 -> MinMax/2, Add4/2
  Ks_shaft [Nm/rad]/1 -> Add2/1, MinMax/1, Add4/1

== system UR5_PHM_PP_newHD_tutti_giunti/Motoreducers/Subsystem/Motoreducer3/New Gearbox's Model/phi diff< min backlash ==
  In2 : Inport
  In3 : Inport  Port=2
  Action Port : ActionPort  PropagateVarSize=During execution  ActionPortLabel=elseif( u2<u4)
  Add1 : Sum  Inputs=+|-
  Add2 : Sum  Inputs=+|+
  Add4 : Sum  Inputs=+|+
  Compare To Zero : simulink/Logic and Bit Operations/Compare To Zero  relop=>=  OutDataTypeStr=uint8
  Constant : Constant  Value=0
  Constant1 : Constant  Value=0
  Cs_shaft [Nm/(rad/s)] : Gain  Gain=J3.C
  Ks_shaft [Nm/rad] : Gain  Gain=J3.K
  MinMax : MinMax  Function=max  Inputs=2
  Switch : Switch  Criteria=u2 > Threshold
  Out1 : Outport  VectorParamsAs1DForOutWhenUnconnected=off
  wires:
  Switch/1 -> Out1/1
  Add2/1 -> Switch/3
  MinMax/1 -> Add2/2
  Add4/1 -> Compare To Zero/1
  Constant/1 -> Switch/1
  Compare To Zero/1 -> Switch/2
  Add1/1 -> Ks_shaft [Nm/rad]/1
  Constant1/1 -> Add1/2
  In2/1 -> Add1/1
  In3/1 -> Cs_shaft [Nm/(rad/s)]/1
  Cs_shaft [Nm/(rad/s)]/1 -> MinMax/2, Add4/2
  Ks_shaft [Nm/rad]/1 -> Add2/1, MinMax/1, Add4/1

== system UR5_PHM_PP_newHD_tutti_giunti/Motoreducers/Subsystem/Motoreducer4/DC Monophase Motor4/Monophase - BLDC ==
  Vset : Inport
  qdm : Inport  Port=2
  Phase A : Subsystem
  Torque constant [Nm/A] : Gain  Gain=Motor.kc_4
  T : Outport  VectorParamsAs1DForOutWhenUnconnected=off
  i : Outport  Port=2  VectorParamsAs1DForOutWhenUnconnected=off
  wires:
  Vset/1 -> Phase A/1(Vset)
  Torque constant [Nm/A]/1 -> T/1
  Phase A/1(i) -> Torque constant [Nm/A]/1, i/1
  qdm/1 -> Phase A/2(qdm)

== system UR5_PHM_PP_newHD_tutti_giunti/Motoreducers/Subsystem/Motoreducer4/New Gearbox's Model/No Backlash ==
  qm : Inport
  q : Inport  Port=2
  qdm : Inport  Port=3
  qd : Inport  Port=4
  Action Port : ActionPort  PropagateVarSize=During execution  ActionPortLabel=if(u1<=1e-10)
  Circular spline : Subsystem
  Flexspline (rad) : Subsystem
  Flexspline (tang) : Subsystem
  Wave Generator : Subsystem
  Ccs->giunto : Outport
  Cwg->rotore : Outport  Port=2
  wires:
  Flexspline (rad)/2(x2) -> Circular spline/3(x2), Flexspline (tang)/2(x2)
  Flexspline (rad)/1(y2) -> Circular spline/2(y2), Flexspline (tang)/1(y2)
  q/1 -> Circular spline/4(q)
  qd/1 -> Circular spline/5(qd)
  Circular spline/1(C1) -> Ccs->giunto/1
  Circular spline/2(q_CS) -> Flexspline (rad)/3(q_CS)
  qm/1 -> Wave Generator/1(qm)
  qdm/1 -> Wave Generator/2(qdm)
  Flexspline (rad)/3(C_FS->WG) -> Wave Generator/3(C_FS->WG)
  Wave Generator/1(qm_WG) -> Flexspline (rad)/1(qm_WG)
  Wave Generator/2(Cwg->rotore) -> Cwg->rotore/1
  Wave Generator/3(qdm_WG) -> Flexspline (rad)/2(qdm_WG)
  Flexspline (tang)/1(y1) -> Flexspline (rad)/4(y1), Circular spline/1(y1)

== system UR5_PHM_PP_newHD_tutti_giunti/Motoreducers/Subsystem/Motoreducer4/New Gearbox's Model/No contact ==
  In2 : Inport
  In3 : Inport  Port=2
  Action Port : ActionPort  PropagateVarSize=During execution  ActionPortLabel=else
  1/(2-1/eta_dir) : Gain  Gain=0
  Add4 : Sum  Inputs=+|+
  Out3 : Outport  VectorParamsAs1DForOutWhenUnconnected=off
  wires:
  Add4/1 -> 1/(2-1/eta_dir)/1
  In3/1 -> Add4/2
  In2/1 -> Add4/1
  1/(2-1/eta_dir)/1 -> Out3/1

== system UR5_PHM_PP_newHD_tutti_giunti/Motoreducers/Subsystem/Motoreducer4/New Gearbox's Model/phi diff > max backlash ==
  In2 : Inport
  In3 : Inport  Port=2
  Action Port : ActionPort  PropagateVarSize=During execution  ActionPortLabel=elseif(u2>u3)
  Add1 : Sum  Inputs=+|-
  Add2 : Sum  Inputs=+|+
  Add4 : Sum  Inputs=+|+
  Compare To Zero : simulink/Logic and Bit Operations/Compare To Zero  relop=<=  OutDataTypeStr=uint8
  Constant : Constant  Value=0
  Constant3 : Constant  Value=J4.clearance
  Cs_shaft [Nm/(rad/s)] : Gain  Gain=J4.C
  Ks_shaft [Nm/rad] : Gain  Gain=J4.K
  MinMax : MinMax  Inputs=2
  Switch : Switch  Criteria=u2 > Threshold
  Out1 : Outport  VectorParamsAs1DForOutWhenUnconnected=off
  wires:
  Switch/1 -> Out1/1
  Add2/1 -> Switch/3
  MinMax/1 -> Add2/2
  Add4/1 -> Compare To Zero/1
  Constant/1 -> Switch/1
  Compare To Zero/1 -> Switch/2
  Add1/1 -> Ks_shaft [Nm/rad]/1
  Constant3/1 -> Add1/2
  In2/1 -> Add1/1
  In3/1 -> Cs_shaft [Nm/(rad/s)]/1
  Cs_shaft [Nm/(rad/s)]/1 -> MinMax/2, Add4/2
  Ks_shaft [Nm/rad]/1 -> Add2/1, MinMax/1, Add4/1

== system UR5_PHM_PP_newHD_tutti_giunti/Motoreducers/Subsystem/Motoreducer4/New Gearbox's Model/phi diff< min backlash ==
  In2 : Inport
  In3 : Inport  Port=2
  Action Port : ActionPort  PropagateVarSize=During execution  ActionPortLabel=elseif( u2<u4)
  Add1 : Sum  Inputs=+|-
  Add2 : Sum  Inputs=+|+
  Add4 : Sum  Inputs=+|+
  Compare To Zero : simulink/Logic and Bit Operations/Compare To Zero  relop=>=  OutDataTypeStr=uint8
  Constant : Constant  Value=0
  Constant1 : Constant  Value=0
  Cs_shaft [Nm/(rad/s)] : Gain  Gain=J4.C
  Ks_shaft [Nm/rad] : Gain  Gain=J4.K
  MinMax : MinMax  Function=max  Inputs=2
  Switch : Switch  Criteria=u2 > Threshold
  Out1 : Outport  VectorParamsAs1DForOutWhenUnconnected=off
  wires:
  Switch/1 -> Out1/1
  Add2/1 -> Switch/3
  MinMax/1 -> Add2/2
  Add4/1 -> Compare To Zero/1
  Constant/1 -> Switch/1
  Compare To Zero/1 -> Switch/2
  Add1/1 -> Ks_shaft [Nm/rad]/1
  Constant1/1 -> Add1/2
  In2/1 -> Add1/1
  In3/1 -> Cs_shaft [Nm/(rad/s)]/1
  Cs_shaft [Nm/(rad/s)]/1 -> MinMax/2, Add4/2
  Ks_shaft [Nm/rad]/1 -> Add2/1, MinMax/1, Add4/1

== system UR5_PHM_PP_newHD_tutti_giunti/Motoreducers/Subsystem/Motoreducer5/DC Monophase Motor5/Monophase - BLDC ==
  Vset : Inport
  qdm : Inport  Port=2
  Phase A : Subsystem
  Torque constant [Nm/A] : Gain  Gain=Motor.kc_5
  T : Outport  VectorParamsAs1DForOutWhenUnconnected=off
  i : Outport  Port=2  VectorParamsAs1DForOutWhenUnconnected=off
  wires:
  Vset/1 -> Phase A/1(Vset)
  Torque constant [Nm/A]/1 -> T/1
  Phase A/1(i) -> Torque constant [Nm/A]/1, i/1
  qdm/1 -> Phase A/2(qdm)

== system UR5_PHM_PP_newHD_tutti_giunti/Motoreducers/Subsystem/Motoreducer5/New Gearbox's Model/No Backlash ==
  qm : Inport
  q : Inport  Port=2
  qdm : Inport  Port=3
  qd : Inport  Port=4
  Action Port : ActionPort  PropagateVarSize=During execution  ActionPortLabel=if(u1<=1e-10)
  Circular spline : Subsystem
  Flexspline (rad) : Subsystem
  Flexspline (tang) : Subsystem
  Wave Generator : Subsystem
  Ccs->giunto : Outport
  Cwg->rotore : Outport  Port=2
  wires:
  Flexspline (rad)/2(x2) -> Circular spline/3(x2), Flexspline (tang)/2(x2)
  Flexspline (rad)/1(y2) -> Circular spline/2(y2), Flexspline (tang)/1(y2)
  Flexspline (tang)/1(y1) -> Flexspline (rad)/4(y1), Circular spline/1(y1)
  q/1 -> Circular spline/4(q)
  qd/1 -> Circular spline/5(qd)
  Circular spline/1(C1) -> Ccs->giunto/1
  Circular spline/2(q_CS) -> Flexspline (rad)/3(q_CS)
  qm/1 -> Wave Generator/1(qm)
  qdm/1 -> Wave Generator/2(qdm)
  Flexspline (rad)/3(C_FS->WG) -> Wave Generator/3(C_FS->WG)
  Wave Generator/1(Cwg->rotore) -> Cwg->rotore/1
  Wave Generator/2(qm_WG) -> Flexspline (rad)/1(qm_WG)
  Wave Generator/3(qdm_WG) -> Flexspline (rad)/2(qdm_WG)

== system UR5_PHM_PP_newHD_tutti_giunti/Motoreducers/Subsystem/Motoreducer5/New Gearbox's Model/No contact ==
  In2 : Inport
  In3 : Inport  Port=2
  Action Port : ActionPort  PropagateVarSize=During execution  ActionPortLabel=else
  1/(2-1/eta_dir) : Gain  Gain=0
  Add4 : Sum  Inputs=+|+
  Out3 : Outport  VectorParamsAs1DForOutWhenUnconnected=off
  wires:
  Add4/1 -> 1/(2-1/eta_dir)/1
  In3/1 -> Add4/2
  In2/1 -> Add4/1
  1/(2-1/eta_dir)/1 -> Out3/1
